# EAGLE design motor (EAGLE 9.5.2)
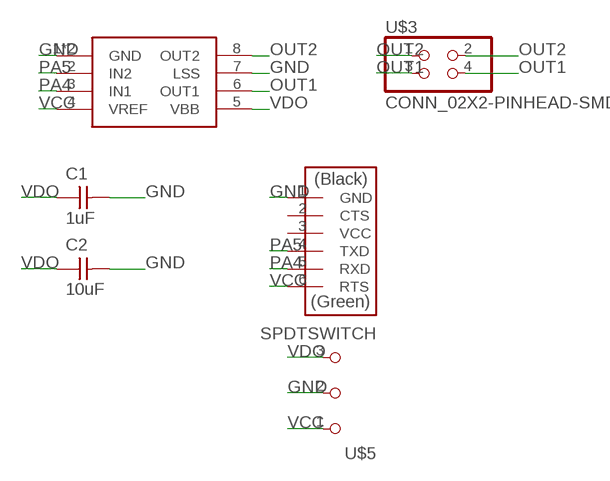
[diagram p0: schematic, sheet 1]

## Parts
C1  1uF  CAP_UNPOLARIZEDFAB  [C1206FAB]
C2  10uF  CAP_UNPOLARIZEDFAB  [C1206FAB]
U$1  CONN_06_FTDI-SMD-HEADER  [1X06SMD]
U$2  PMIC_H-BRIDGE_A4953_PAD  [SOIC8_PAD]
U$3  CONN_02X2-PINHEAD-SMD  [2X02SMD]
U$5  SPDTSWITCH  [SPDTSWITCH]

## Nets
GND: C1.2 C2.2 U$1.1(GND) U$2.1(GND) U$2.7(LSS) U$2.GND U$5.2
OUT1: U$2.6(OUT1) U$3.3 U$3.4
OUT2: U$2.8(OUT2) U$3.1 U$3.2
PA4: U$1.5(RXD) U$2.3(IN1)
PA5: U$1.4(TXD) U$2.2(IN2)
VCC: U$1.6(RTS) U$2.4(VREF) U$5.1
VDO: C1.1 C2.1 U$2.5(VBB) U$5.3
Unconnected: U$1.2(CTS) U$1.3(VCC)

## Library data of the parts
C1 C2 = fab:CAP_UNPOLARIZED
U$1 = fab:CONN_06_FTDI-SMD-HEADER
U$2 = fab:PMIC_H-BRIDGE_A4953_PAD
U$3 = fab:CONN_02X2-PINHEAD-SMD
U$5 = fab:SPDTSWITCH

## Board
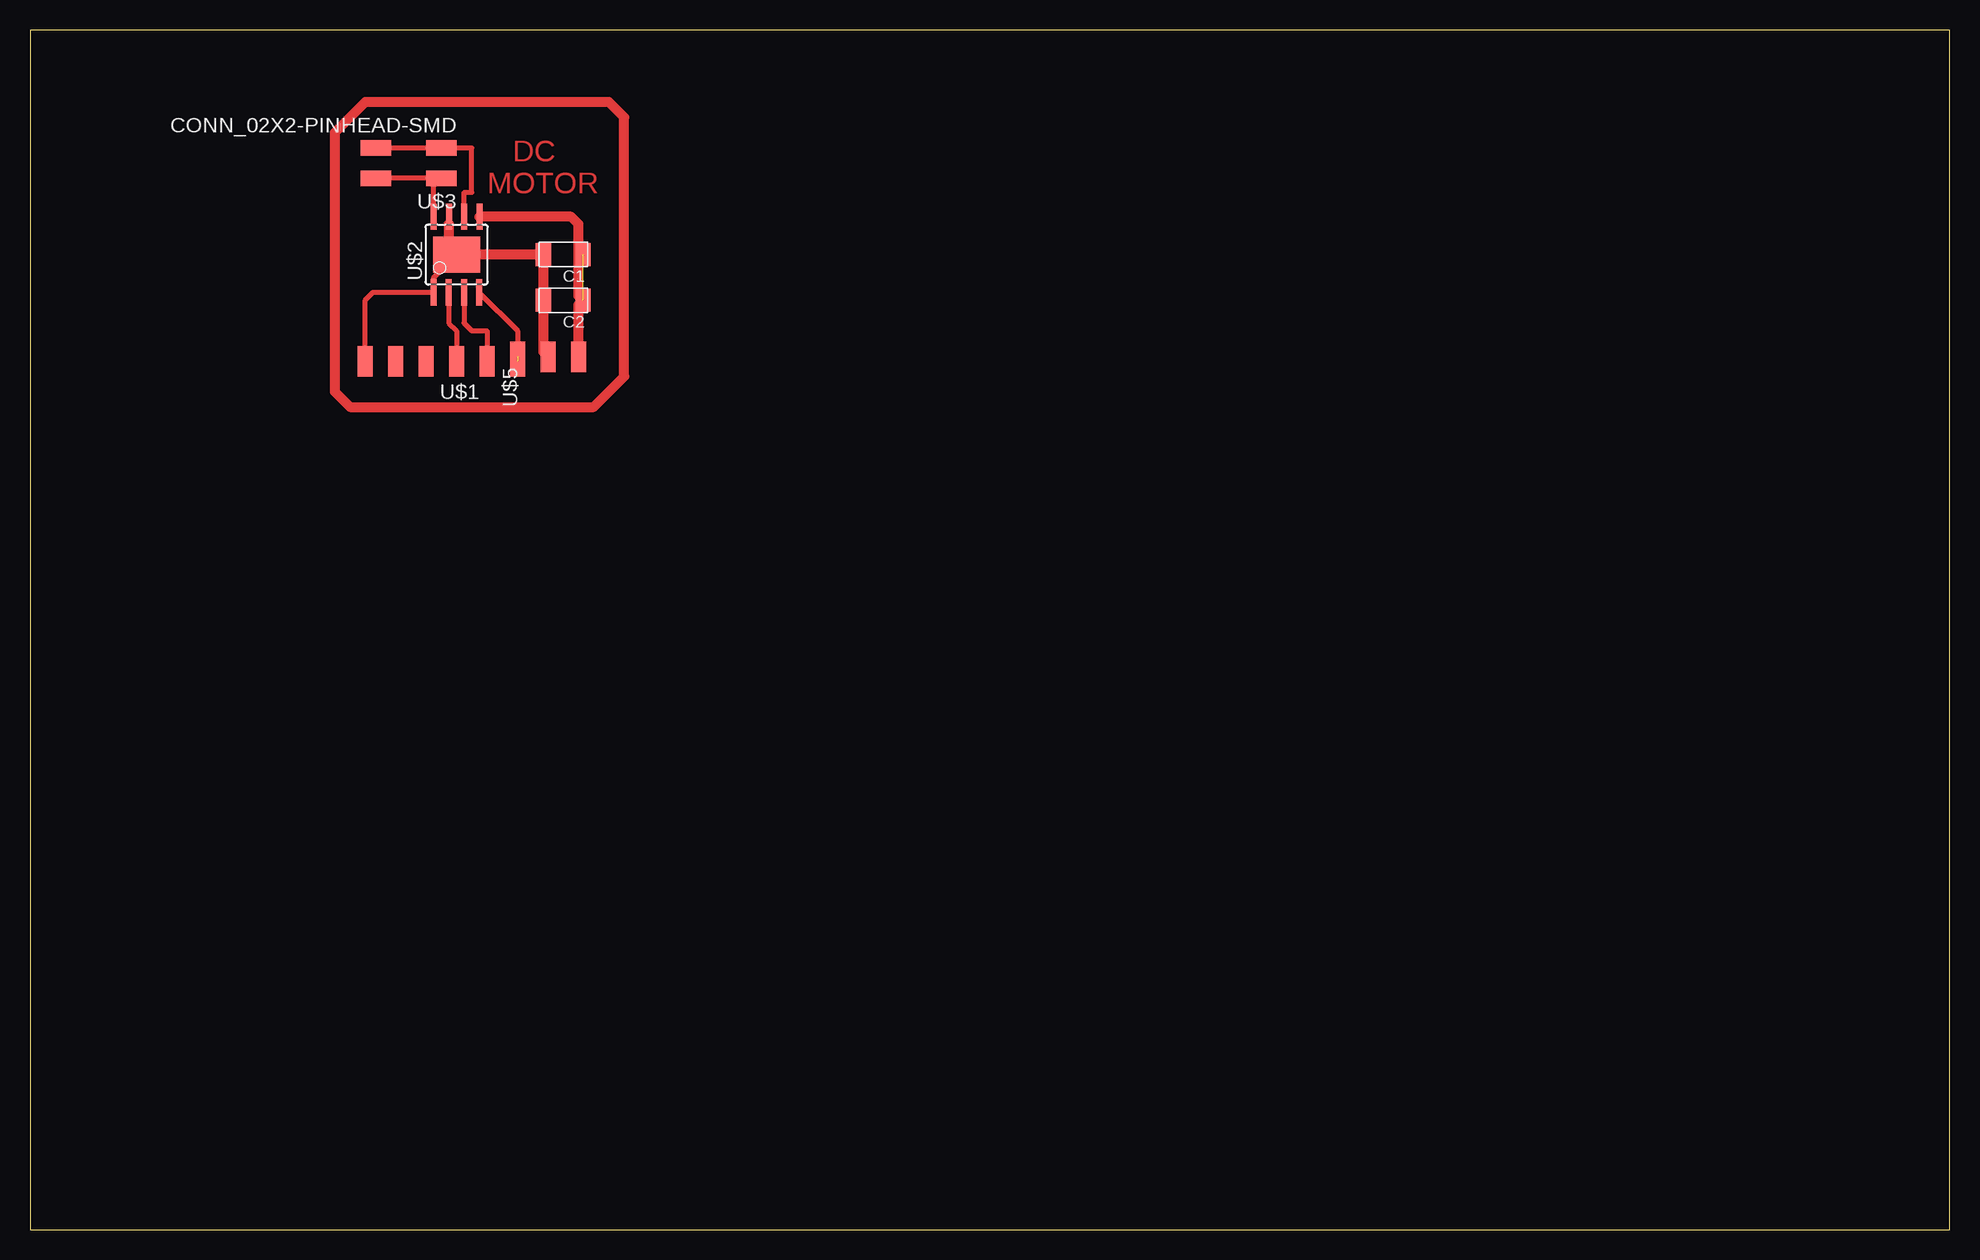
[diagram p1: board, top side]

Size 160 x 100 mm. Coordinates in mm from the lower left corner, seen from the top.
Outline: 0,0 160,0 160,100 0,100 0,0
Copper layers (1*16): Top 0.035mm / dielectric 1.5mm / Bottom 0.035mm
Design rules "default": minimum track width 6mil, minimum drill 0.35mm, track to track 6mil, track to pad 6mil, pad to pad 6mil, via to via 6mil, smd to smd 6mil, copper to edge 40mil, drill to drill 6mil, minimum pad ring 10mil, minimum via ring 8mil, stop-mask expansion 4mil, vias tented up to drill 0mil, thermal gap 10mil

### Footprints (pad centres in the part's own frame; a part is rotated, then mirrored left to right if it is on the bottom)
C1206FAB = smd 1.27 x 1.905: 1 -1.651,0; 2 1.651,0
1X06SMD = smd 2.54 x 1.27: 1 0,6.35; 2 0,3.81; 3 0,1.27; 4 0,-1.27; 5 0,-3.81; 6 0,-6.35
SOIC8_PAD = smd 0.5 x 2.2: 1 -1.905,-3.154; 2 -0.645,-3.154; 3 0.625,-3.154; 4 1.895,-3.154; 5 1.905,3.154; 6 0.635,3.154; 7 -0.635,3.154; 8 -1.905,3.154 | smd 3.886 x 2.997: GND 0,0
2X02SMD = smd 2.54 x 1.27: 1 -2.54,1.27; 2 2.92,1.27; 3 -2.54,-1.27; 4 2.92,-1.27
SPDTSWITCH = smd 2.54 x 1.27: 1 0.38,2.54; 2 0.38,0; 3 0.38,-2.54

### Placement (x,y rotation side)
C1  44.45,81.28 180 top
C2  44.45,77.47 180 top
U$1  34.29,72.39 90 top
U$2  35.56,81.28 0 top
U$3  31.75,88.9 180 top
U$5  43.18,72.39 90 top

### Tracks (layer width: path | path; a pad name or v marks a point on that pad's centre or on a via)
GND
  Top 0.406: U$1.1 27.94,77.47 28.6,78.13 U$2.1 33.66,79.38 34.92,80.64 34.92,81.28 34.92,83.82 U$2.7
  Top 0.813: U$5.2 42.8,73.15 C2.2 C1.2 34.92,81.28 | U$2.GND 34.92,81.92 34.92,83.82
N$1
  Top 0.813: 25.4,91.44 25.4,69.85 26.67,68.58 46.99,68.58 49.53,71.12 49.53,92.71 48.26,93.98 27.94,93.98 25.4,91.44
OUT1
  Top 0.406: U$3.4 U$3.3 36.83,90.17 36.83,86.47 36.2,86.47 U$2.6
OUT2
  Top 0.406: U$2.8 33.66,87 U$3.1 U$3.2
PA4
  Top 0.406: U$2.3 36.19,75.58 36.83,74.93 38.1,74.93 U$1.5
PA5
  Top 0.406: U$2.2 34.91,75.58 35.56,74.93 U$1.4
VCC  (1 unrouted)
  Top 0.406: U$2.4 37.45,78.11 40.64,74.93 U$5.1
VDO  (1 unrouted)
  Top 0.813: U$5.3 45.72,77.09 C2.1 45.72,77.85 45.72,83.82 45.11,84.43 U$2.5

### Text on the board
Top: DC / MOTOR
